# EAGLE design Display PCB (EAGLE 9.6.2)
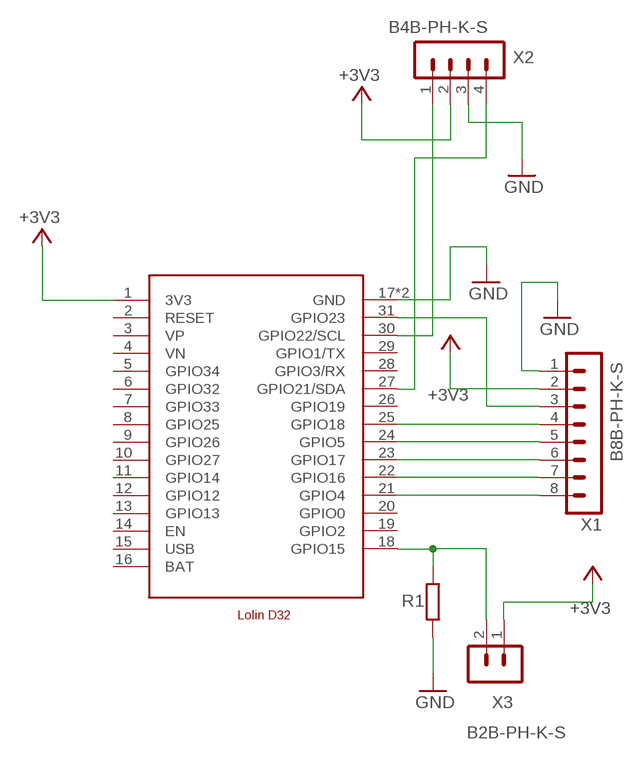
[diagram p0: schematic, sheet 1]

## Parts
R1  R-EU_R0805  [R0805]
U$1  LOLIND32  [LOLIND32]
X1  B8B-PH-K-S  [B8B-PH-K-S]
X2  B4B-PH-K-S  [B4B-PH-K-S]
X3  B2B-PH-K-S  [B2B-PH-K-S]

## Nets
+3V3: U$1.1(3V3) X1.2 X2.2 X3.1
BUSY: U$1.21(GPIO4) X1.8
CLK: U$1.25(GPIO18) X1.4
CS: U$1.24(GPIO5) X1.5
DC: U$1.23(GPIO17) X1.6
DIN: U$1.31(GPIO23) X1.3
GND: R1.1 U$1.17(GND) U$1.32(GND) X1.1 X2.3
N$9: R1.2 U$1.18(GPIO15) X3.2
RST: U$1.22(GPIO16) X1.7
SCL: U$1.30(GPIO22/SCL) X2.1
SDA: U$1.27(GPIO21/SDA) X2.4
Unconnected: U$1.2(RESET) U$1.3(VP) U$1.4(VN) U$1.5(GPIO34) U$1.6(GPIO32) U$1.7(GPIO33) U$1.8(GPIO25) U$1.9(GPIO26) U$1.10(GPIO27) U$1.11(GPIO14) U$1.12(GPIO12) U$1.13(GPIO13) U$1.14(EN) U$1.19(GPIO2) U$1.20(GPIO0) U$1.26(GPIO19) U$1.28(GPIO3/RX) U$1.29(GPIO1/TX)

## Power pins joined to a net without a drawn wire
BAT: U$1.16(BAT)
USB: U$1.15(USB)

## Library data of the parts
R1 = rcl:R-EU_: RESISTOR, European symbol; SPICEPREFIX: R
U$1 = microcontroller:LOLIND32: Wemos Lolin D32 Lolin D32 is a development board based on ESP32. On this schematic, this board is designed with battery port. Pins VP and VN are Not Connected pins.
X1 = con-JSTPH:B8B-PH: JST PH series header 2.00mm pitch disconnectable crimp style connectors, vertical (side entry type), 8 pins
X2 = con-JSTPH:B4B-PH: JST PH series header 2.00mm pitch disconnectable crimp style connectors, vertical (side entry type), 4 pins
X3 = con-JSTPH:B2B-PH: JST PH series header 2.00mm pitch disconnectable crimp style connectors, vertical (side entry type), 2 pins

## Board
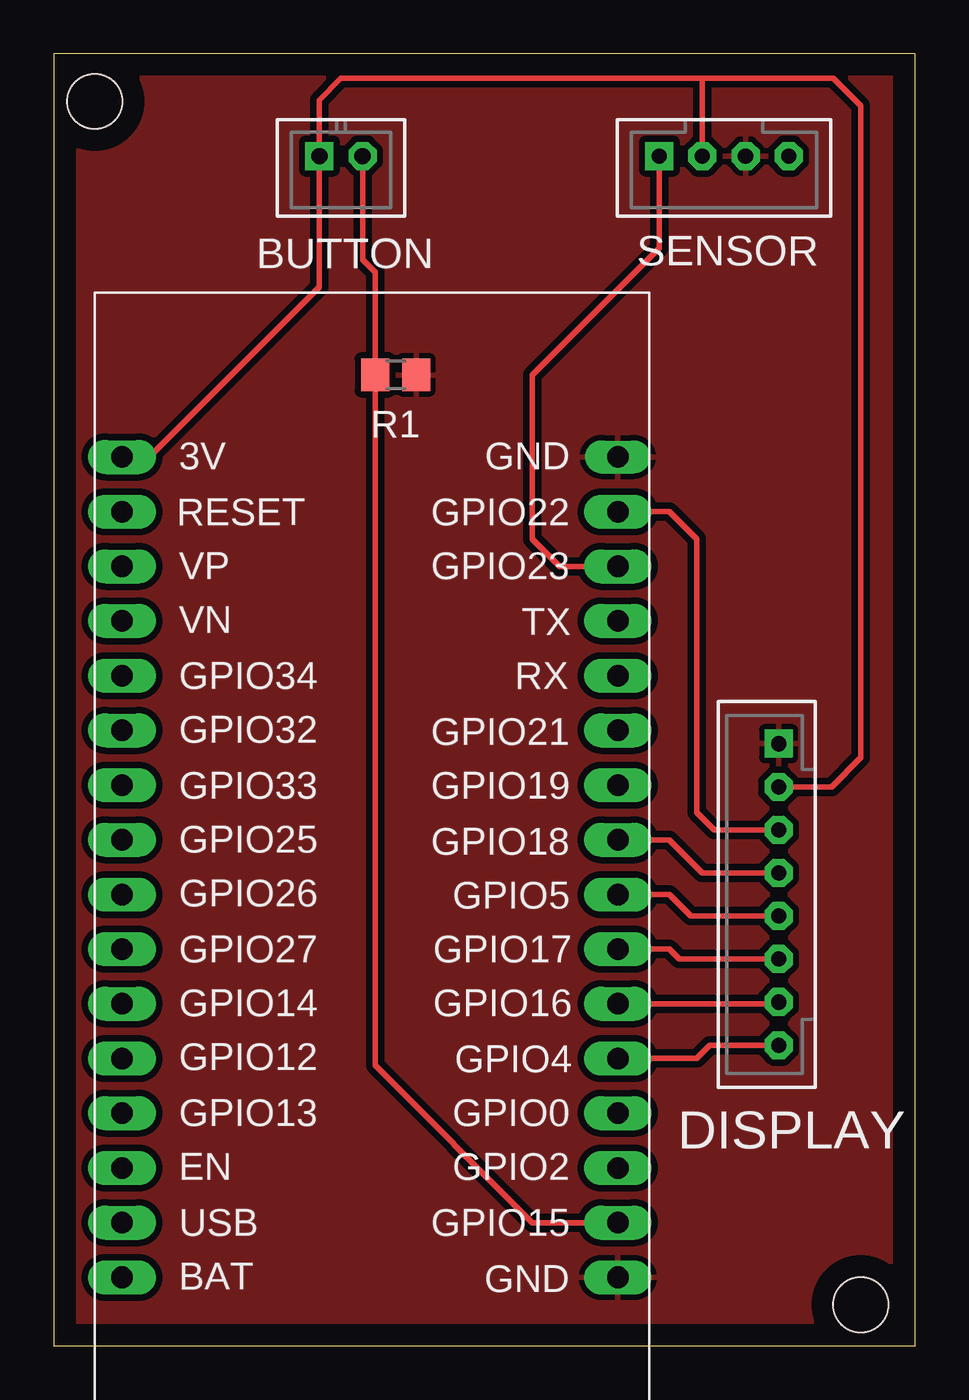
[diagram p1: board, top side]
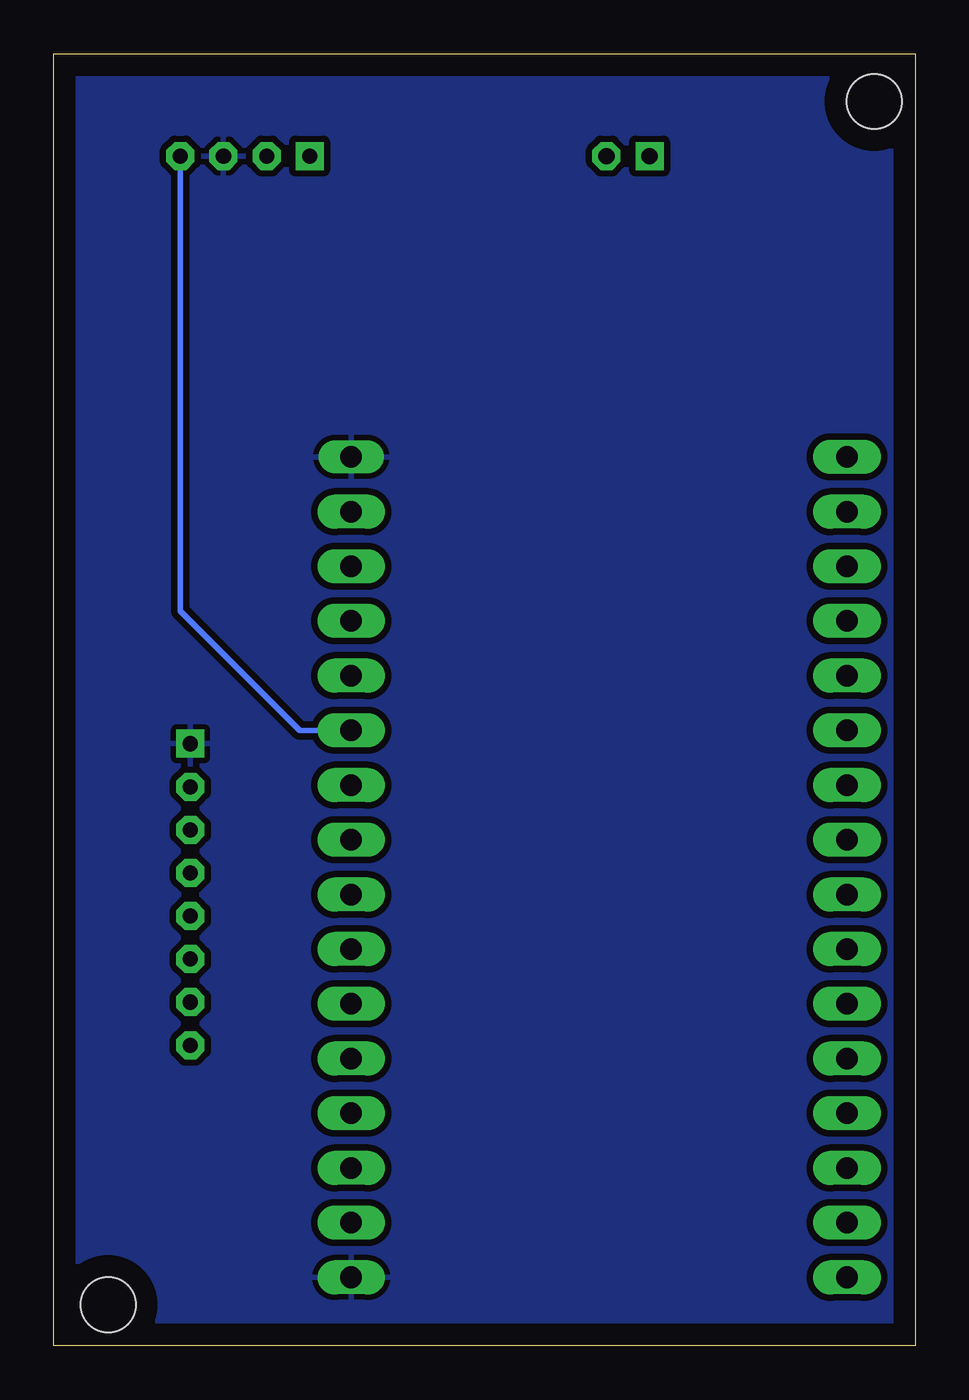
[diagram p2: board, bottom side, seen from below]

Size 39.98 x 60 mm. Coordinates in mm from the lower left corner, seen from the top.
Outline: 0,0 39.98,0 39.98,60 0,60 0,0
Copper layers (1*16): Top 0.035mm / dielectric 1.5mm / Bottom 0.035mm
Design rules "default": minimum track width 6mil, minimum drill 0.35mm, track to track 6mil, track to pad 6mil, pad to pad 6mil, via to via 6mil, smd to smd 6mil, copper to edge 40mil, drill to drill 6mil, minimum pad ring 10mil, minimum via ring 8mil, stop-mask expansion 4mil, vias tented up to drill 0mil, thermal gap 10mil
Holes 2.54 mm at 1.9,57.79 37.46,1.91

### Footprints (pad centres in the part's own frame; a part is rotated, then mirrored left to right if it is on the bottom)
R0805 = smd 1.3 x 1.5: 1 -0.95,0; 2 0.95,0
LOLIND32 = drill 1 pad 1.575 long: 1 -11.43,21.59; 2 -11.43,19.05; 3 -11.43,16.51; 4 -11.43,13.97; 5 -11.43,11.43; 6 -11.43,8.89; 7 -11.43,6.35; 8 -11.43,3.81; 9 -11.43,1.27; 10 -11.43,-1.27; 11 -11.43,-3.81; 12 -11.43,-6.35; 13 -11.43,-8.89; 14 -11.43,-11.43; 15 -11.43,-13.97; 16 -11.43,-16.51; 17 11.58,-16.51; 18 11.58,-13.97; 19 11.58,-11.43; 20 11.58,-8.89; 21 11.58,-6.35; 22 11.58,-3.81; 23 11.58,-1.27; 24 11.58,1.27; 25 11.58,3.81; 26 11.58,6.35; 27 11.58,8.89; 28 11.58,11.43; 29 11.58,13.97; 30 11.58,16.51; 31 11.58,19.05 | drill 1 pad 1.524 long: 32 11.58,21.59
B8B-PH-K-S = drill 0.7 pad 1.3 square: 1 7,0 | drill 0.7 pad 1.3 octagon: 2 5,0; 3 3,0; 4 1,0; 5 -1,0; 6 -3,0; 7 -5,0; 8 -7,0
B4B-PH-K-S = drill 0.7 pad 1.3 square: 1 3,0 | drill 0.7 pad 1.3 octagon: 2 1,0; 3 -1,0; 4 -3,0
B2B-PH-K-S = drill 0.75 pad 1.3 square: 1 1,0 | drill 0.75 pad 1.3 octagon: 2 -1,0

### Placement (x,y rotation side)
R1  15.87,45.09 180 top
U$1  14.6,19.68 0 top
X1  33.65,20.96 90 top
X2  31.11,55.25 180 top
X3  13.33,55.25 180 top

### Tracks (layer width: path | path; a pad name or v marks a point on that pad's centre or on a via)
+3V3
  Top 0.254: U$1.1 4.44,41.28 12.33,49.17 X3.1 12.33,57.85 13.33,58.85 30.11,58.85 | X1.2 36.11,25.96 37.46,27.31 37.46,57.58 36.19,58.85 30.11,58.85 | X2.2 30.11,58.85
BUSY
  Top 0.254: X1.8 30.46,13.96 29.84,13.34 U$1.21
CLK
  Top 0.254: X1.4 30.11,21.96 28.57,23.5 U$1.25
CS
  Top 0.254: X1.5 29.57,19.96 28.57,20.96 U$1.24
DC
  Top 0.254: X1.6 29.03,17.96 28.57,18.42 U$1.23
DIN
  Top 0.254: X1.3 30.65,23.96 29.84,24.77 29.84,37.47 28.57,38.73 U$1.31
GND
  pour Top (isolate 0.305): -0.64,-0.63 40,-0.63 40,60.33 -0.64,60.33
  pour Bottom (isolate 0.305): -0.64,60.33 40,60.33 40,-0.63 -0.64,-0.63
N$9
  Top 0.254: U$1.18 22.22,5.71 14.92,13.02 R1.2 14.92,49.84 14.33,50.44 X3.2
RST
  Top 0.254: X1.7 33.57,15.88 U$1.22
SCL
  Top 0.254: X2.1 28.11,50.98 22.22,45.09 22.22,37.47 23.49,36.2 U$1.30
SDA
  Bottom 0.254: X2.4 34.11,34.12 28.57,28.57 U$1.27

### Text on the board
tPlace: BUTTON | SENSOR | DISPLAY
